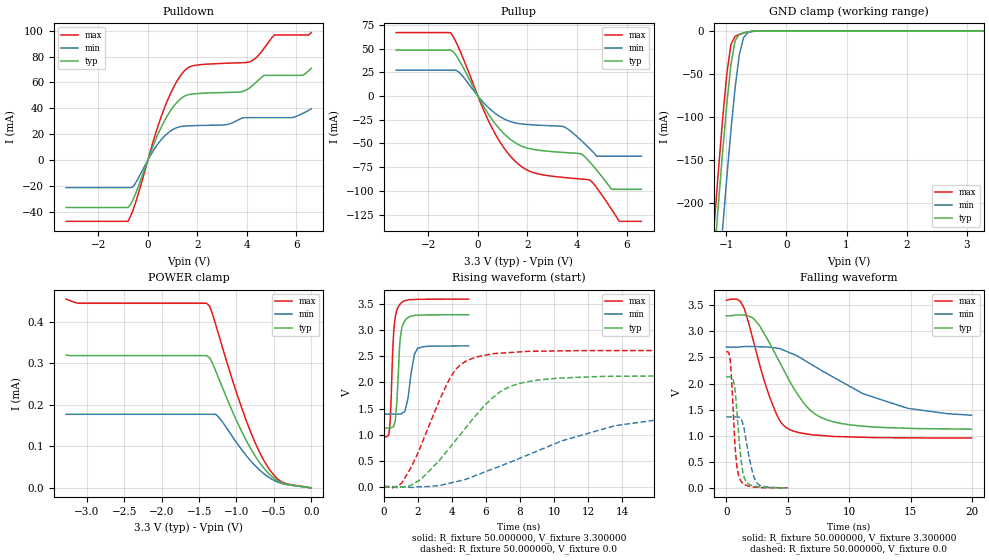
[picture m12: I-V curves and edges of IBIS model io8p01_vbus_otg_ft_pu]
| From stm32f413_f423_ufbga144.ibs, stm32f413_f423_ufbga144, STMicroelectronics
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|   Model io8p01_vbus_otg_ft_pu
[Model]  io8p01_vbus_otg_ft_pu
Model_type I/O
Polarity   Non-Inverting
Enable   Active-Low
Vinl =   0.990000V
Vinh =   2.310000V
Vmeas =  1.650000V
Cref =   50.000000pF
Rref =   100.000000M
Vref =   0.0V
C_comp   3.304800pF   3.199300pF   3.429300pF
[Temperature Range]   25.000000   0.125000k   -40.000000
[Pullup Reference]   3.300000V   2.700000V   3.600000V
[Pulldown Reference]   0.0V   0.0V   0.0V
[POWER Clamp Reference]   3.300000V   2.700000V   3.600000V
[GND Clamp Reference]   0.0V   0.0V   0.0V
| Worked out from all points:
|   slope of the pulldown table from 0 to 0.495 V, typ, clamps not added: 20.9 ohm
|   slope of the pullup table from 0 to 0.495 V, typ, clamps not added: 22.6 ohm
|   GND clamp passes 1 mA (typ) near -0.61 V on its own axis
|   rising waveform, R_fixture 50.000000, V_fixture 3.300000: 20-80 % time 224ps typ, 350ps min, 206ps max; typ from 1.12 V to 3.3 V
|   rising waveform, R_fixture 50.000000, V_fixture 0.0: 20-80 % time 3.36ns typ, 6.84ns min, 2.08ns max; typ from 0.001 V to 2.13 V
|   falling waveform, R_fixture 50.000000, V_fixture 3.300000: 20-80 % time 3.23ns typ, 6.66ns min, 2.03ns max; typ from 3.3 V to 1.12 V
|   falling waveform, R_fixture 50.000000, V_fixture 0.0: 20-80 % time 481ps typ, 679ps min, 387ps max; typ from 2.13 V to 0.001 V
[Pulldown]
|Voltage   I(typ)   I(min)   I(max)
-3.3V     -36.41mA   -21.08mA   -47.04mA
-800mV    -36.41mA   -21.08mA   -47.04mA
-600mV    -30.48mA   -20.53mA   -38.65mA
700mV     31.4mA     19.11mA    41.71mA
1.2V      45.15mA    25.37mA    61.75mA
1.6V      50.35mA    26.5mA     71.06mA
3.1V      52.28mA    27.26mA    74.76mA
4.1V      55.64mA    32.87mA    75.8mA
4.7V      65.47mA    32.87mA    86.49mA
5.1V      65.47mA    32.87mA    96.56mA
6.2V      65.47mA    35.57mA    96.56mA
6.6V      70.92mA    39.71mA    98.46mA
[Pullup]
|Voltage   I(typ)   I(min)   I(max)
-3.3V     48.4mA     27.38mA    66.91mA
-1.1V     48.4mA     27.38mA    66.69mA
-700mV    35.09mA    23.45mA    46.29mA
500mV     -22.06mA   -14mA      -30.03mA
1.5V      -49.1mA    -28.3mA    -68.56mA
2.2V      -56.04mA   -30.32mA   -80.35mA
3.5V      -59.52mA   -32.65mA   -85.91mA
4.5V      -69.06mA   -55.12mA   -88.39mA
4.8V      -78.22mA   -63.4mA    -96.84mA
5.4V      -98.3mA    -63.4mA    -119.6mA
5.7V      -98.3mA    -63.4mA    -132mA
6.6V      -98.3mA    -63.4mA    -132mA
[GND_clamp]
|Voltage   I(typ)   I(min)   I(max)
-3.3V     -2.321A    -2.399A    -2.294A
-1.2V     -265.6mA   -356.2mA   -227.3mA
-1.13V    -202.8mA   -293mA     -164.3mA
-1.06V    -142.3mA   -231.2mA   -104.3mA
-990mV    -86.15mA   -171.7mA   -51mA
-920mV    -39.05mA   -115.6mA   -15.71mA
-850mV    -11.4mA    -65.74mA   -6.366mA
-780mV    -4.046mA   -27.6mA    -4.153mA
-710mV    -2.285mA   -7.882mA   -2.591mA
-640mV    -1.291mA   -2.274mA   -1.367mA
-570mV    -618uA     -909.9uA   -567.3uA
3.28V     0A         0A         0A
[POWER_clamp]
|Voltage   I(typ)   I(min)   I(max)
-3.28V    319.9uA    177.1uA    454.3uA
-3.12V    318.3uA    177.1uA    444.3uA
-1.4V     318.3uA    177.1uA    444.3uA
-1.36V    313.4uA    177.1uA    437.2uA
-1.28V    282.3uA    177.1uA    394.1uA
-1.24V    264.6uA    170.9uA    369.7uA
-920mV    131.9uA    89.38uA    187.2uA
-760mV    79.47uA    55.16uA    112.7uA
-640mV    48.78uA    35.06uA    68.06uA
-520mV    26.21uA    20.13uA    35uA
-400mV    12.52uA    10.84uA    14.88uA
0V        0A         0A         0A
[Ramp]
| variable   typ   min   max
dV/dt_r  1.27735/3.35408n   0.79905/6.86364n   1.56700/2.07505n
dV/dt_f  1.30152/3.22709n   0.73896/6.63899n   1.58712/2.03241n
R_load = 50.000000
[Rising Waveform]
R_fixture= 50.000000
V_fixture= 3.300000
V_fixture_min= 2.700000
V_fixture_max= 3.600000
|time   V(typ)   V(min)   V(max)
0s        1.125V     1.393V     955.6mV
300.3ps   1.127V     1.393V     1.027V
370.4ps   1.129V     1.393V     1.286V
580.6ps   1.173V     1.393V     2.994V
670.7ps   1.281V     1.393V     3.265V
850.9ps   2.216V     1.394V     3.455V
930.9ps   2.74V      1.395V     3.493V
1.101ns   3.103V     1.416V     3.548V
1.982ns   3.29V      2.657V     3.595V
4.985ns   3.3V       2.7V       3.599V
[Rising Waveform]
R_fixture= 50.000000
V_fixture= 0.0
V_fixture_min= 0.0
V_fixture_max= 0.0
|time   V(typ)   V(min)   V(max)
0s        1.446mV    1.246mV    1.808mV
1.081ns   -5.986mV   -865.8uV   88.76mV
2.162ns   135.8mV    248.7uV    776.8mV
3.804ns   723.2mV    62.24mV    2.033V
4.284ns   917.3mV    99mV       2.271V
4.885ns   1.161V     150.5mV    2.421V
6.807ns   1.816V     392.3mV    2.561V
8.288ns   2.004V     586.1mV    2.593V
13.61ns   2.118V     1.172V     2.612V
19.94ns   2.129V     1.36V      2.612V
[Falling Waveform]
R_fixture= 50.000000
V_fixture= 3.300000
V_fixture_min= 2.700000
V_fixture_max= 3.600000
|time   V(typ)   V(min)   V(max)
0s        3.3V       2.7V       3.599V
1.441ns   3.312V     2.71V      3.444V
2.162ns   3.259V     2.71V      2.851V
3.524ns   2.773V     2.697V     1.742V
4.324ns   2.415V     2.672V     1.301V
5.045ns   2.094V     2.602V     1.132V
6.807ns   1.494V     2.383V     1.024V
8.649ns   1.27V      2.13V      987.5mV
14.73ns   1.143V     1.527V     960.1mV
19.94ns   1.125V     1.393V     955.6mV
[Falling Waveform]
R_fixture= 50.000000
V_fixture= 0.0
V_fixture_min= 0.0
V_fixture_max= 0.0
|time   V(typ)   V(min)   V(max)
0s        2.129V     1.36V      2.612V
300.3ps   2.13V      1.359V     2.477V
620.6ps   2.02V      1.359V     1.199V
810.8ps   1.615V     1.361V     518.7mV
1.111ns   736.1mV    1.345V     164.5mV
1.301ns   356.4mV    1.267V     96.59mV
1.522ns   160.8mV    1.031V     60.57mV
2.142ns   41.55mV    284.9mV    18.51mV
2.452ns   26.28mV    108.8mV    12.68mV
4.985ns   1.446mV    1.246mV    1.808mV
